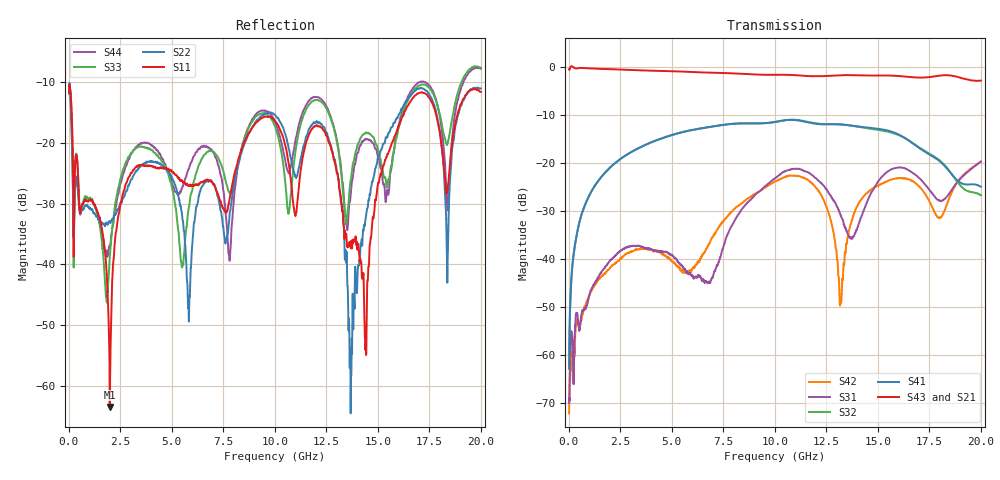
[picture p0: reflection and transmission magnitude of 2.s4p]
!Keysight Technologies,N5225A,MY51451420,A.10.40.12
!Date: Tuesday, October 13, 2015 10:20:25
!Correction: S11(Full 4 Port(1,2,3,4))
!S12(Full 4 Port(1,2,3,4))
!S13(Full 4 Port(1,2,3,4))
!S14(Full 4 Port(1,2,3,4))
!S21(Full 4 Port(1,2,3,4))
!S22(Full 4 Port(1,2,3,4))
!S23(Full 4 Port(1,2,3,4))
!S24(Full 4 Port(1,2,3,4))
!S31(Full 4 Port(1,2,3,4))
!S32(Full 4 Port(1,2,3,4))
!S33(Full 4 Port(1,2,3,4))
!S34(Full 4 Port(1,2,3,4))
!S41(Full 4 Port(1,2,3,4))
!S42(Full 4 Port(1,2,3,4))
!S43(Full 4 Port(1,2,3,4))
!S44(Full 4 Port(1,2,3,4))
!S4P File: Measurements: <S11,S12,S13,S14>,
!<S21,S22,S23,S24>,
!<S31,S32,S33,S34>,
!<S41,S42,S43,S44>:
# Hz S  dB  R 50
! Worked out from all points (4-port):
!   1999 points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, 20 MHz to 20 GHz, reference 50 ohm
!   strongest paths, dB at 20 MHz, 5.01 GHz, 10.01 GHz, 15.01 GHz, 20 GHz:
!     S43: -0.5, -0.9, -1.6, -1.8, -2.8
!     S21: -0.5, -0.9, -1.6, -1.8, -2.3
!     S41: -62.8, -14.2, -11.4, -12.9, -24.9
!     S32: -62.2, -14.1, -11.5, -13.1, -26.7
!     S31: -69.9, -39.2, -23.2, -23.9, -19.7
!     S42: -72.1, -40.4, -23.8, -24.6, -19.7
!   lowest |S11| = -63.5 dB at 1.99 GHz (marker M1), VSWR 1.00, Z = 49.9 - j0.0344 ohm
!   |S11| at or under -10 dB: start of sweep to end of sweep
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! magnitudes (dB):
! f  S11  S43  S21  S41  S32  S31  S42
! 20 MHz  -11.8  -0.5  -0.5  -62.8  -62.2  -69.9  -72.1
! 1.99 GHz  -63.5  -0.4  -0.4  -21.0  -21.0  -40.4  -41.9
! 3.2 GHz  -24.2  -0.6  -0.6  -17.3  -17.3  -37.2  -38.1
! 12.19 GHz  -17.3  -1.9  -1.7  -11.9  -11.8  -23.9  -26.3
! 13.67 GHz  -36.4  -1.7  -1.7  -12.2  -12.2  -35.5  -32.8
! 15.45 GHz  -22.0  -1.8  -1.8  -13.2  -13.4  -21.8  -23.8
! 20 GHz  -11.6  -2.8  -2.3  -24.9  -26.7  -19.7  -19.7
